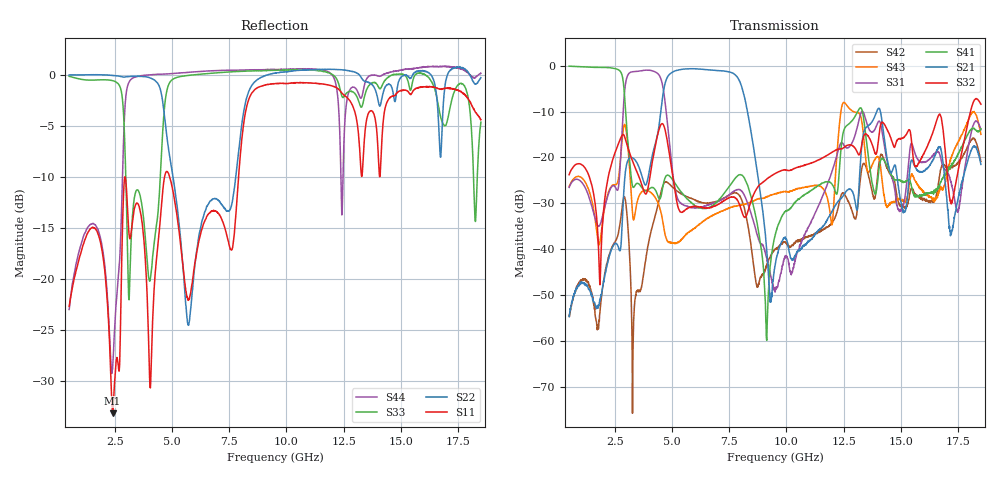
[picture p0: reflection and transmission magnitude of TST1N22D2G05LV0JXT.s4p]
# MHZ S RI R 50
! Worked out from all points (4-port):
!   1801 points, 500 MHz to 18.5 GHz, reference 50 ohm
!   strongest paths, dB at 500 MHz, 5 GHz, 9.5 GHz, 14 GHz, 18.5 GHz:
!     S32: -23.8, -23.1, -23.5, -17.2, -8.4
!     S21: -54.7, -1.4, -43.7, -9.5, -21.5
!     S41: -0.1, -24.7, -37.1, -24.6, -13.7
!     S31: -26.5, -22.3, -49.4, -12.3, -14.0
!     S43: -26.4, -38.8, -28.0, -19.9, -15.0
!     S42: -54.4, -26.4, -40.0, -23.1, -20.9
!   lowest |S11| = -33.2 dB at 2.4 GHz (marker M1), VSWR 1.04, Z = 52.2 - j0.0484 ohm
!   |S11| at or under -10 dB: start of sweep to 2.935 GHz; 2.952 GHz to 4.671 GHz (1.718 GHz wide, 45.1 % of centre); 4.899 GHz to 7.907 GHz (3.008 GHz wide, 47 % of centre)
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500  -0.0285 -0.0677  -0.00129 0.00137  0.035 0.0315  0.9149 -0.3751
     -0.00129 0.00131  0.9651 -0.2757  0.049 0.043  -0.000919 0.00158
     0.0349 0.0316  0.0485 0.043  0.1587 -0.9756  0.0413 0.0243
     0.9161 -0.374  -0.00104 0.00159  0.0414 0.0243  -0.00967 -0.07
1670  -0.1664 0.0533  -0.00111 0.00213  0.0201 -0.00191  0.1675 -0.9455
      -0.00102 0.00209  0.5784 -0.8239  0.013 -0.0236  0.00125 -0.00113
      0.0202 -0.00184  0.0132 -0.0234  -0.1389 0.9375  -0.0137 -0.0123
      0.1669 -0.9465  0.00129 -0.00109  -0.0136 -0.0122  -0.1333 -0.124
2400  0.0219 -0.000463  -0.0105 0.00173  0.0409 0.0267  -0.7108 -0.623
      -0.0104 0.00174  0.1855 -0.9805  0.0719 0.0593  -0.00573 0.00907
      0.041 0.0268  0.0724 0.0595  0.9079 -0.2481  0.0496 -0.00686
      -0.711 -0.6226  -0.00569 0.00911  0.0494 -0.00706  0.0116 -0.0341
5840  0.0342 -0.0828  0.7885 0.4916  -0.0279 0.00508  -0.0106 0.0301
      0.7885 0.4901  0.04 -0.065  0.0262 -0.0122  0.032 -0.0158
      -0.0279 0.00516  0.0262 -0.0121  0.3206 -0.9495  -0.0154 0.00414
      -0.0108 0.0302  0.0321 -0.0159  -0.0155 0.00412  -0.6936 -0.7695
9130  -0.1231 -0.8902  0.00702 0.00749  0.00794 -0.00135  0.000455 0.00092
      0.00696 0.00763  0.7079 -0.7082  -0.0579 0.00396  -0.00578 0.0032
      0.00802 -0.00119  -0.0577 0.00411  -0.8052 -0.6792  -0.0221 0.0292
      0.000563 0.000874  -0.00566 0.00316  -0.0223 0.03  -0.8947 -0.5773
14790  -0.5811 0.5643  -0.0471 0.0565  0.0179 0.0298  0.0473 0.0315
       -0.0488 0.0576  -0.7863 -0.0178  0.0784 0.1227  0.0101 0.0451
       0.0178 0.0297  0.0776 0.1201  -0.4818 0.8906  0.00841 0.0319
       0.0469 0.0324  0.011 0.0422  0.0101 0.0321  -1.035 0.1921
18500  -0.266 0.5436  0.0806 -0.018  0.1219 -0.157  0.1124 0.1687
       0.0811 -0.0213  -0.4288 -0.8734  0.3702 0.0813  0.0826 0.0317
       0.1187 -0.1617  0.3717 0.0829  -0.0117 -0.5881  0.1729 0.0413
       0.119 0.1678  0.0839 0.0335  0.1741 0.0397  -0.822 -0.6088
